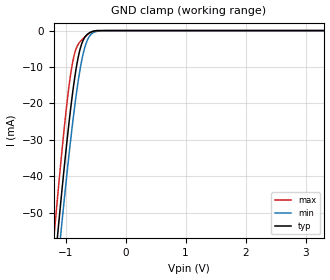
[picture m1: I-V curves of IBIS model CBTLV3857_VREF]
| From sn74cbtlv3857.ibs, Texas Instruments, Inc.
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[Model]   CBTLV3857_VREF
Model_type  Input
Vinl = 1.0
Vinh = 1.33
| variable   typ   min   max
C_comp   2.98pF   2.17pF   3.77pF
[Temperature Range]   40   100   -40
| Ambient temperature   25   85   -40
[Voltage range]   3.3   3   3.6
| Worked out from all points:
|   GND clamp passes 1 mA (typ) near -0.63 V on its own axis
[GND Clamp]
| CBTLV3857_VREF
|   Voltage   I(typ)   I(min)   I(max)
-3.3V     -485.3mA   -483.2mA   -490.7mA
-1.19V    -66.45mA   -74.91mA   -56.19mA
-1.125V   -54.98mA   -63.67mA   -44.36mA
-1.085V   -48.1mA    -56.91mA   -37.34mA
-1.07V    -45.57mA   -54.41mA   -34.77mA
-955mV    -27.22mA   -36.03mA   -16.95mA
-865mV    -15.02mA   -23.12mA   -7.389mA
-745mV    -4.366mA   -9.479mA   -2.808mA
-670mV    -1.628mA   -4.136mA   -1.625mA
-590mV    -511.7uA   -1.312mA   -609.3uA
-355mV    -1.584uA   -26.33uA   -23.29nA
3.3V      1.153nA    59.69nA    33.43pA
